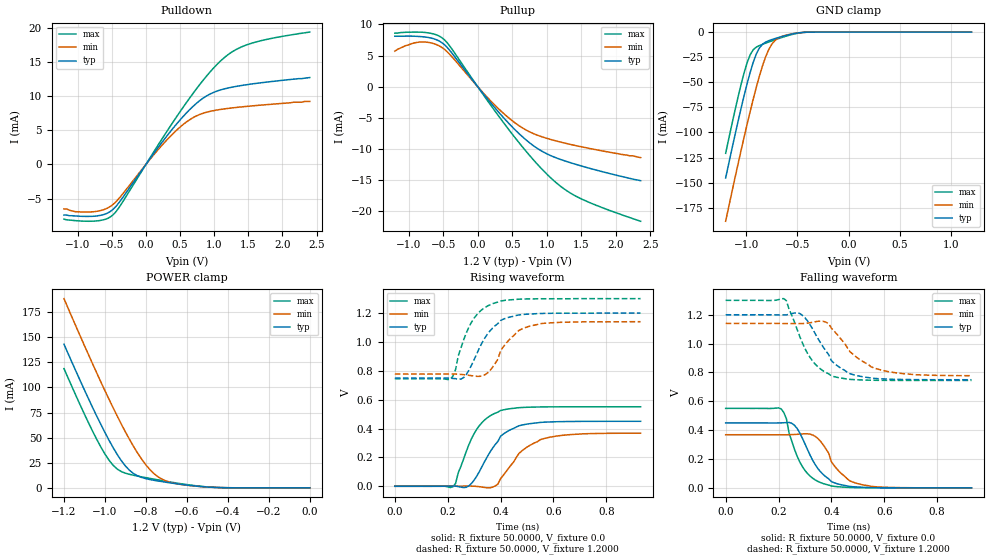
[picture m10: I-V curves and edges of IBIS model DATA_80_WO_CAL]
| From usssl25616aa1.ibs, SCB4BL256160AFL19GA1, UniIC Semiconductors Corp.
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|   Model DATA_80_WO_CAL
[Model]  DATA_80_WO_CAL
Model_type I/O
Polarity   Non-Inverting
Enable   Active-High
Vinl =   0.3800V
Vinh =   0.8200V
Vmeas =  0.6000V
Cref =   5.0000pF
Rref =   50.0000
Vref =   0.6000V
C_comp   1.7430pF   1.7110pF   1.7640pF
[Temperature Range]   25.0000   0.1250k   -40.0000
[Voltage Range]   1.2000V   1.1400V   1.3000V
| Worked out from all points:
|   slope of the pulldown table from 0 to 0.18 V, typ, clamps not added: 72.3 ohm
|   slope of the pullup table from 0 to 0.18 V, typ, clamps not added: 72.5 ohm
|   GND clamp passes 1 mA (typ) near -0.50 V on its own axis
|   POWER clamp passes 1 mA (typ) near -0.51 V on its own axis
|   rising waveform, R_fixture 50.0000, V_fixture 0.0: 20-80 % time 93.1ps typ, 113ps min, 85.6ps max; typ from 0 V to 0.45 V
|   rising waveform, R_fixture 50.0000, V_fixture 1.2000: 20-80 % time 87.8ps typ, 83ps min, 75.5ps max; typ from 0.75 V to 1.2 V
|   falling waveform, R_fixture 50.0000, V_fixture 0.0: 20-80 % time 84.5ps typ, 83.4ps min, 71ps max; typ from 0.45 V to 0 V
|   falling waveform, R_fixture 50.0000, V_fixture 1.2000: 20-80 % time 102ps typ, 123ps min, 87.9ps max; typ from 1.2 V to 0.75 V
[Pulldown]
|Voltage   I(typ)   I(min)   I(max)
-1.2V     -7.4mA     -6.5mA     -8mA
-1.04V    -7.53mA    -6.9mA     -8.21mA
-760mV    -7.573mA   -6.91mA    -8.293mA
-600mV    -7.269mA   -6.543mA   -8.036mA
-480mV    -6.557mA   -5.837mA   -7.359mA
-360mV    -5.125mA   -4.557mA   -5.782mA
200mV     2.759mA    2.402mA    3.175mA
520mV     6.727mA    5.628mA    7.998mA
840mV     9.703mA    7.488mA    12.33mA
1.2V      11.16mA    8.184mA    16.02mA
1.6V      11.83mA    8.596mA    17.87mA
2.4V      12.7mA     9.2mA      19.35mA
[Pullup]
|Voltage   I(typ)   I(min)   I(max)
-1.2V     8.1mA      5.7mA      8.6mA
-1.04V    8.11mA     6.6mA      8.73mA
-840mV    8.05mA     7.16mA     8.75mA
-680mV    7.819mA    7.032mA    8.569mA
-520mV    7.078mA    6.309mA    7.875mA
-400mV    5.766mA    5.134mA    6.459mA
120mV     -1.673mA   -1.484mA   -1.9mA
440mV     -5.77mA    -4.931mA   -6.744mA
760mV     -9.09mA    -7.301mA   -11.15mA
1.08V     -11.18mA   -8.55mA    -14.87mA
1.48V     -12.67mA   -9.61mA    -17.91mA
2.36V     -15.1mA    -11.4mA    -21.62mA
[GND_clamp]
|Voltage   I(typ)   I(min)   I(max)
-1.2V     -145.3mA   -188.5mA   -120.8mA
-1.05V    -76.2mA    -118.2mA   -52.43mA
-990mV    -51.2mA    -91.62mA   -30.39mA
-960mV    -39.9mA    -78.82mA   -22.48mA
-900mV    -21.67mA   -54.7mA    -15mA
-870mV    -15.78mA   -43.66mA   -13.45mA
-810mV    -10.04mA   -24.79mA   -11.07mA
-780mV    -8.658mA   -17.59mA   -9.958mA
-720mV    -6.57mA    -8.545mA   -7.793mA
-630mV    -3.906mA   -3.64mA    -4.741mA
-420mV    -215.4uA   -240.5uA   -235uA
1.2V      1.597nA    22.84nA    1.463nA
[POWER_clamp]
|Voltage   I(typ)   I(min)   I(max)
-1.2V     143mA      188.4mA    118.7mA
-1.1V     97.38mA    141.5mA    73.24mA
-1.04V    71.38mA    114.3mA    48.22mA
-1V       55.04mA    96.69mA    33.64mA
-960mV    40mA       79.65mA    22.42mA
-900mV    21.75mA    55.6mA     14.58mA
-860mV    14.17mA    41.05mA    12.52mA
-800mV    9.133mA    22.79mA    10.12mA
-740mV    6.786mA    10.88mA    7.886mA
-660mV    4.332mA    4.436mA    5.101mA
-520mV    1.103mA    1.063mA    1.274mA
0V        1.597nA    6.003nA    2.16nA
[Ramp]
| variable   typ   min   max
dV/dt_r  0.2701/95.9095p   0.2207/0.1140n   0.3305/79.6325p
dV/dt_f  0.2703/0.1038n   0.2174/0.1267n   0.3332/81.7811p
R_load = 50.0000
[Rising Waveform]
R_fixture= 50.0000
V_fixture= 0.0
V_fixture_min= 0.0
V_fixture_max= 0.0
|time   V(typ)   V(min)   V(max)
0s        0V         0V         0V
220ps     1.302mV    165.9uV    -3.005mV
230ps     1.356mV    303.7uV    20.35mV
270ps     -7.188mV   1.252mV    239.7mV
310ps     69.87mV    -947.9uV   395.1mV
370ps     264.3mV    -6.071mV   497.7mV
400ps     346.6mV    52.37mV    524.9mV
470ps     419.3mV    228.1mV    544.6mV
550ps     442.3mV    322.8mV    549.5mV
930ps     450.1mV    367.9mV    550.8mV
[Rising Waveform]
R_fixture= 50.0000
V_fixture= 1.2000
V_fixture_min= 1.1400
V_fixture_max= 1.3000
|time   V(typ)   V(min)   V(max)
0s        749.5mV    777.1mV    744.6mV
210ps     748.3mV    777.7mV    740.6mV
230ps     745.3mV    777.4mV    809.4mV
260ps     752.1mV    773.2mV    1.012V
300ps     876.7mV    763.5mV    1.165V
350ps     1.053V     783.8mV    1.248V
400ps     1.148V     938.4mV    1.283V
470ps     1.187V     1.08V      1.296V
550ps     1.197V     1.126V     1.299V
930ps     1.2V       1.14V      1.3V
[Falling Waveform]
R_fixture= 50.0000
V_fixture= 0.0
V_fixture_min= 0.0
V_fixture_max= 0.0
|time   V(typ)   V(min)   V(max)
0s        450.1mV    368.1mV    550.8mV
210ps     450.5mV    367.7mV    547.6mV
230ps     452.6mV    367.8mV    478.1mV
250ps     447.6mV    369.1mV    324.7mV
290ps     344.9mV    373.8mV    148.1mV
330ps     188.6mV    365.7mV    65.62mV
370ps     90.71mV    296mV      28.97mV
420ps     29.49mV    132.7mV    8.486mV
500ps     5.41mV     28.88mV    1.344mV
930ps     748nV      9.655uV    0V
[Falling Waveform]
R_fixture= 50.0000
V_fixture= 1.2000
V_fixture_min= 1.1400
V_fixture_max= 1.3000
|time   V(typ)   V(min)   V(max)
0s        1.2V       1.14V      1.3V
220ps     1.199V     1.139V     1.312V
230ps     1.199V     1.139V     1.297V
290ps     1.197V     1.139V     1.006V
340ps     1.065V     1.152V     855.4mV
380ps     947.4mV    1.148V     798.9mV
400ps     882.1mV    1.107V     776.3mV
470ps     791.7mV    944.9mV    752mV
560ps     759.1mV    832.3mV    745.8mV
930ps     749.5mV    777.6mV    744.6mV
